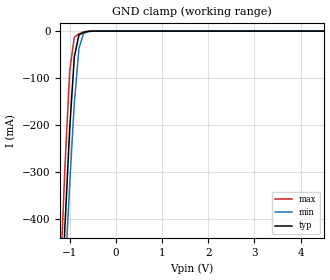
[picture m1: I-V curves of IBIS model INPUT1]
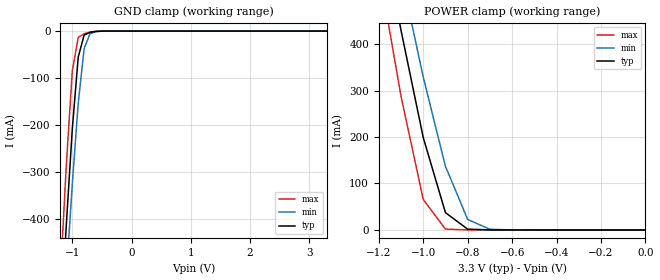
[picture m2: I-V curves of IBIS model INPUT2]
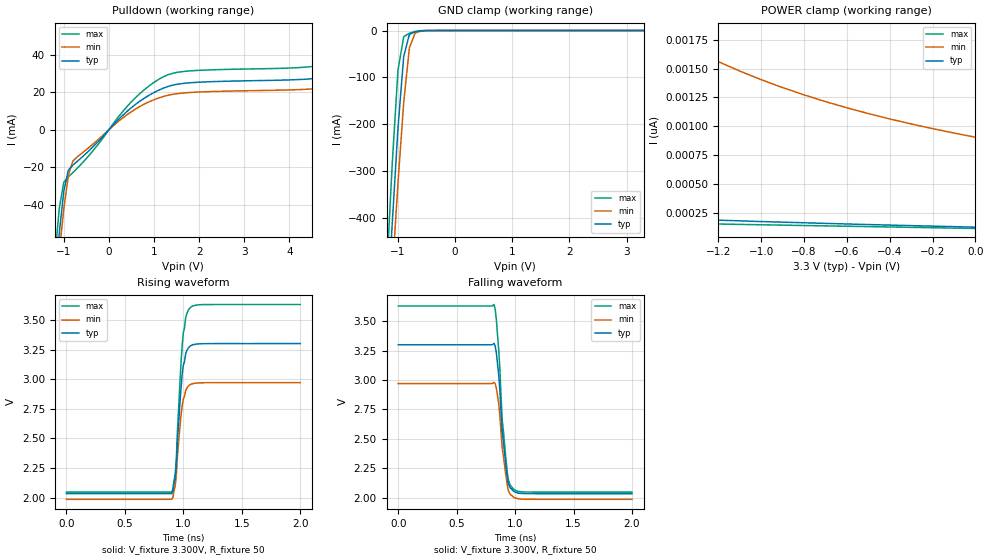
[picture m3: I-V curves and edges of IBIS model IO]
|   PERICOM SEMICONDUCTOR CORP
|   IBIS Model of PI6CFGL201B
|   Product Family: 6CFGL
|   24 Pin (ZD)TQFN Package
[IBIS Ver] 3.2
[Comment char] |_char
[File Name] pi6cfgl201b_zd_reva.ibs
[File Rev] 1.0
[Source] File originated at Pericom Semiconductor Corp.
[Date] 6/14/2017
[Disclaimer] (C) Copyright PERICOM Semiconductor Corporation
   All rights reserved
  Pericom Semiconductor Corporation hereby grants the user of
  this IBIS model a non-exclusive, nontransferable license to
  use this IBIS model under the following terms.
  This IBIS model is provided on an "AS IS" basis and Pericom
  makes absolutely no warranty with respect to the information
  contained herein. PERICOM DISCLAIMS AND CUSTOMER WAIVES ALL
  WARRANTIES, EXPRESSED OR IMPLIED, INCLUDING WARRANTIES OF
  MERCHANTABILITY OR FITNESS FOR A PARTICULAR PURPOSE. The
  entire risk as to quality and performance is with the customer.
  Accordingly, in no event shall the company be liable for any
  damages, whether in contract or tort, including any lost
  profits or other incidental, consequential, exemplary, or
  punitive damages arising out of the use or application of the
  IBIS model provided in this package. Further, Pericom reserves
  the right to make changes without notice to any product herein
  to improve reliability, function, or design. Pericom does not
  convey any license under patent rights or any other intellectual
  property rights, including those of third parties.
  The user is granted this license only to use the IBIS model
  and is not granted rights to sell, load, rent, lease or license
  the IBIS model in whole or in part, or in modified form to anyone
  other than user. User may modify the IBIS model to suit its specific
  application but rights to derivative works and such modifications
  shall belong to Pericom.
  Pericom is not obligated to provide maintenance or support
  for the licensed IBIS model.
  Contact Pericom at ATTN: APPLICATION ENGINEERING / IBIS MODELS
  Milpitas, CA 95134
[Component] PI6CFGL201B
[Manufacturer] Pericom Semiconductor Corp.
[Package]
|   typ   min   max
R_pkg   0.03484ohm   0.02922ohm   0.04046ohm
L_pkg   0.78416nH   0.76828nH   0.80005nH
C_pkg   0.18668pF   0.17176pF   0.20160pF
[Pin]   signal_name   model_name   R_pin   L_pin   C_pin
1   XTAL_IN   INPUT1   0.04046   0.80005nH   0.20160pF
2   XTAL_OUT   NC   0.03484   0.78416nH   0.18668pF
3   VDDXTAL   POWER   0.02922   0.76828nH   0.17176pF
4   SADR/REF18   NC   0.02922   0.76828nH   0.17176pF
5   VDDREF18   POWER   0.03484   0.78416nH   0.18668pF
6   GNDDIG   GND   0.04046   0.80005nH   0.20160pF
7   VDDDIG33   POWER   0.04046   0.80005nH   0.20160pF
8   SCLK_33   INPUT2   0.03484   0.78416nH   0.18668pF
9   SDATA_33   IO   0.02922   0.76828nH   0.17176pF
10   GND   GND   0.02922   0.76828nH   0.17176pF
11   VDDO18   POWER   0.03484   0.78416nH   0.18668pF
12   OE0#   INPUT2   0.04046   0.80005nH   0.20160pF
13   CLK0   OUTPUT   0.04046   0.80005nH   0.20160pF
14   CLK0#   OUTPUT   0.03484   0.78416nH   0.18668pF
15   GNDA   GND   0.02922   0.76828nH   0.17176pF
16   VDDA33   POWER   0.02922   0.76828nH   0.17176pF
17   CLK1   OUTPUT   0.03484   0.78416nH   0.18668pF
18   CLK1#   OUTPUT   0.04046   0.80005nH   0.20160pF
19   OE1#   INPUT2   0.04046   0.80005nH   0.20160pF
20   VDDO18   POWER   0.03484   0.78416nH   0.18668pF
21   GND   GND   0.02922   0.76828nH   0.17176pF
22   CKPWRGD_PD#   NC   0.02922   0.76828nH   0.17176pF
23   SS_EN_tri   NC   0.03484   0.78416nH   0.18668pF
24   GNDXTAL   GND   0.04046   0.80005nH   0.20160pF
[Diff Pin] inv_pin  vdiff   tdelay_typ  tdelay_min   tdelay_max
13   14   NA   NA   NA   NA
17   18   NA   NA   NA   NA
| Models and submodels in the file (4): INPUT1 (Input), INPUT2 (Input), IO (I/O_open_drain), OUTPUT (Output)
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|   Model INPUT1
[Model] INPUT1
Model_type Input
Vinl = 990mV
Vinh = 2.31V
| variable   typ   min   max
C_comp   1.20pF   1.10pF   1.30pF
[Voltage Range]   3.30V   2.97V   3.63V
[GND Clamp Reference]   0.00V   0.00V   0.00V
[POWER Clamp Reference]  3.30V   2.97V   3.63V
[temperature range]   25   85   -40
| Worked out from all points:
|   GND clamp passes 1 mA (typ) near -0.62 V on its own axis
[GND Clamp]
| Voltage   I(typ)   I(min)  I(max)
-3.3V     -5.593A    -5.259A    -6.024A
-1.2V     -630.5mA   -723.1mA   -521.5mA
-1.1V     -410.9mA   -519.6mA   -283.6mA
-1V       -208.6mA   -326.1mA   -85.11mA
-900mV    -55.41mA   -153.8mA   -13.13mA
-800mV    -8.363mA   -36.98mA   -5.824mA
-700mV    -2.776mA   -5.256mA   -1.937mA
-600mV    -668.6uA   -1.177mA   -276.1uA
-500mV    -76.74uA   -202.8uA   -15.54uA
6.6V      461.1pA    8.82nA     211.8pA
[POWER Clamp]   |Note: Vtable = Vcc - Voutput
| Voltage   I(typ)   I(min)   I(max)
-3.3V     0A         0A         0A
0V        0A         0A         0A
|   Model INPUT2
[Model] INPUT2
Model_type Input
Vinl = 990mV
Vinh = 2.31V
| variable   typ   min   max
C_comp   1.20pF   1.10pF   1.30pF
[Voltage Range]   3.30V   2.97V   3.63V
[GND Clamp Reference]   0.00V   0.00V   0.00V
[POWER Clamp Reference]  3.30V   2.97V   3.63V
[temperature range]   25   85   -40
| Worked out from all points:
|   GND clamp passes 1 mA (typ) near -0.62 V on its own axis
|   POWER clamp passes 1 mA (typ) near -0.75 V on its own axis
[GND Clamp]
| Voltage   I(typ)   I(min)   I(max)
-3.3V     -5.593A    -5.259A    -6.024A
-1.2V     -630.5mA   -723.1mA   -521.5mA
-1.1V     -410.9mA   -519.6mA   -283.6mA
-1V       -208.6mA   -326.1mA   -85.11mA
-900mV    -55.41mA   -153.8mA   -13.13mA
-800mV    -8.363mA   -36.98mA   -5.824mA
-700mV    -2.776mA   -5.256mA   -1.937mA
-600mV    -668.6uA   -1.177mA   -276.1uA
-500mV    -76.74uA   -202.8uA   -15.54uA
3.3V      127.4pA    1.034nA    105.7pA
[POWER Clamp]   |Note: Vtable = Vcc - Voutput
| Voltage   I(typ)   I(min)   I(max)
-3.3V     6.395A     6.003A     6.903A
-1.2V     683.2mA    786.5mA    562.5mA
-1.1V     429.6mA    551.3mA    287.7mA
-1V       198.8mA    329.1mA    65.63mA
-900mV    37.2mA     136.9mA    1.914mA
-800mV    1.74mA     22.66mA    149.1uA
-700mV    141.8uA    1.49mA     13.46uA
0V        127.6pA    905.9pA    116.1pA
|   Model IO
[Model]  IO
Model_type I/O_open_drain
Vinl = 990mV
Vinh = 2.31V
Vref=3.300V
Vmeas=2.5V
Rref=50
|Variable   typ   min   max
C_comp   0.8p   0.7p   0.9p
[Voltage Range]   3.30V   2.97V   3.63V
[Temperature Range]   25   85   -40
[Pulldown Reference]   0.00V   0.00V   0.00V
[Power Clamp Reference]   3.30V   2.97V   3.63V
[GND Clamp Reference]   0.00V   0.00V   0.00V
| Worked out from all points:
|   slope of the pulldown table from 0 to 0.495 V, typ, clamps not added: 42.4 ohm
|   GND clamp passes 1 mA (typ) near -0.62 V on its own axis
|   rising waveform, V_fixture 3.300V, R_fixture 50: 20-80 % time 50.5ps typ, 50.5ps min, 51ps max; typ from 2.03 V to 3.3 V
|   falling waveform, V_fixture 3.300V, R_fixture 50: 20-80 % time 60ps typ, 59.4ps min, 62.8ps max; typ from 3.3 V to 2.03 V
[GND Clamp]
| Voltage   I(typ)   I(min)  I(max)
-3.3V     -5.593A    -5.259A    -6.024A
-1.2V     -630.5mA   -723.1mA   -521.5mA
-1.1V     -410.9mA   -519.6mA   -283.6mA
-1V       -208.6mA   -326.1mA   -85.11mA
-900mV    -55.41mA   -153.8mA   -13.13mA
-800mV    -8.363mA   -36.98mA   -5.824mA
-700mV    -2.776mA   -5.256mA   -1.937mA
-600mV    -668.6uA   -1.177mA   -276.1uA
-500mV    -76.74uA   -202.8uA   -15.54uA
3.3V      127.4pA    1.034nA    105.7pA
[POWER Clamp]
| Voltage   I(typ)   I(min)  I(max)
-3.3V     461.2pA    6.81nA     223.2pA
-2.9V     375.1pA    4.983nA    209.4pA
-2.5V     310.7pA    3.672nA    196.7pA
-2V       251.7pA    2.561nA    180.6pA
-1.5V     208.7pA    1.853nA    163.9pA
-1.4V     201.5pA    1.747nA    160.8pA
-1.3V     194.4pA    1.649nA    157.9pA
-1.1V     182.1pA    1.479nA    151.2pA
-800mV    165.3pA    1.273nA    141.6pA
-600mV    154.9pA    1.161nA    135.4pA
-400mV    145.3pA    1.064nA    129pA
0V        127.4pA    905.9pA    116.1pA
[Pulldown]
| Voltage   I(typ)   I(min)  I(max)
-3.3V     -700mA     -664.7mA   -753.9mA
-1.2V     -81.07mA   -90.27mA   -68.43mA
-1.1V     -54.85mA   -65.19mA   -41.82mA
-1V       -32.74mA   -42.19mA   -27.94mA
-900mV    -21.63mA   -24.34mA   -25.11mA
-800mV    -18.85mA   -16.74mA   -22.83mA
500mV     11.77mA    9.629mA    14.9mA
1.2V      22.07mA    17.66mA    28.1mA
1.8V      25mA       19.82mA    31.33mA
5V        28.54mA    22.91mA    35.47mA
5.8V      33.8mA     27.3mA     42.24mA
6.6V      44.62mA    36.26mA    55.89mA
[Rising Waveform]
V_fixture = 3.300V
V_fixture_min = 2.970V
V_fixture_max = 3.630V
R_fixture = 50
|   Time   V(typ)   V(min)   V(max)
0s        2.033V     1.985V     2.046V
900ps     2.033V     1.985V     2.046V
930ps     2.162V     2.094V     2.196V
940ps     2.273V     2.186V     2.326V
950ps     2.48V      2.354V     2.572V
980ps     2.918V     2.692V     3.135V
1ns       3.116V     2.832V     3.392V
1.03ns    3.241V     2.924V     3.552V
1.07ns    3.285V     2.959V     3.612V
2ns       3.3V       2.97V      3.63V
[Falling Waveform]
V_fixture = 3.300V
V_fixture_min = 2.970V
V_fixture_max = 3.630V
R_fixture = 50
|   Time   V(typ)   V(min)   V(max)
0s        3.3V       2.97V      3.63V
820ps     3.312V     2.98V      3.643V
840ps     3.228V     2.929V     3.509V
860ps     3.042V     2.799V     3.257V
870ps     2.904V     2.695V     3.083V
890ps     2.554V     2.419V     2.659V
930ps     2.203V     2.128V     2.246V
950ps     2.099V     2.042V     2.125V
990ps     2.052V     2.002V     2.07V
2ns       2.033V     1.985V     2.046V
[Ramp]
| variable   typ   min   max
dV/dt_r  0.7603/54.873p   0.5909/55.411p   0.9502/54.771p
dV/dt_f  0.7603/52.221p   0.5910/51.469p   0.9502/54.003p
R_load = 50.0000
